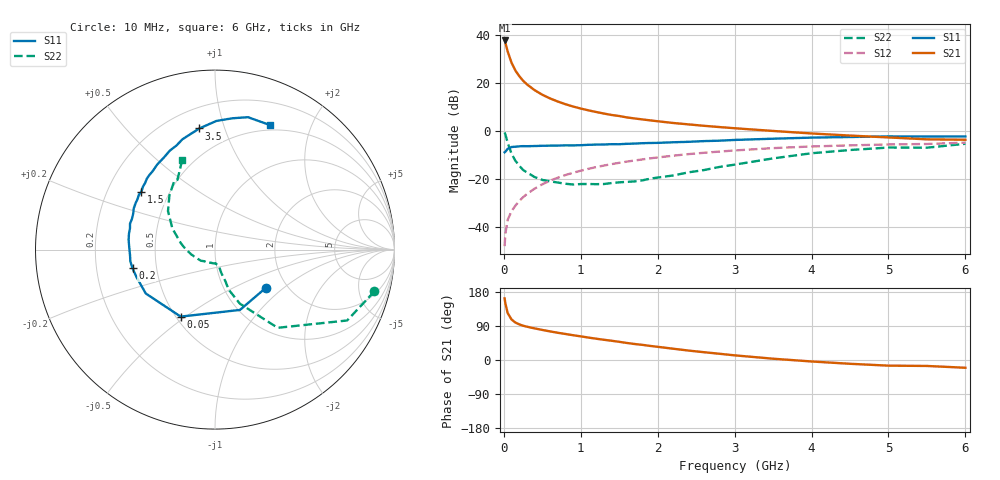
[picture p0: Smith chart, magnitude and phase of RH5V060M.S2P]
! SIEMENS Small Signal Semiconductors
! BFR106
! Si NPN RF Bipolar Junction Transistor in SOT23
! VCE = 5 V  IC = 60 mA
! Common Emitter S-Parameters:  August  1996
# GHz  S  MA  R  50
!  f  S11  S21  S12  S22
! GHz  MAG  ANG  MAG  ANG  MAG  ANG  MAG  ANG
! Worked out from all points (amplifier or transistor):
!   36 points, 10 MHz to 6 GHz, reference 50 ohm
!   highest |S21| = 37.6 dB at 10 MHz (marker M1)
!   |S21| within 3 dB of that: start of sweep to 36.78 MHz
!   unconditionally stable (mu >= 1): 234.5 MHz to 2.299 GHz
!   at 250 MHz: K = 1.01, MAG = 23.6 dB, |S12| = -27.8 dB
!   at 1.4 GHz: K = 1.05, MAG = 8.8 dB, |S12| = -14.0 dB
!   at 6 GHz: K = 0.99, MSG = 0.6 dB, |S12| = -5.0 dB
!   S11 on the Smith chart (normalised r, x): 10 MHz: 1.56, -0.76; 50 MHz: 0.53, -0.48; 200 MHz: 0.36, -0.10; 1.5 GHz: 0.35, +0.31; 3.5 GHz: 0.33, +0.82; 6 GHz: 0.44, +1.44
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0.01  0.3543 -37.0  76.22 162.7  0.0039 83.4  0.9181 -14.7
0.02  0.3638 -67.5  68.27 149.2  0.0072 71.1  0.8356 -28.2
0.05  0.4194 -117.1  44.83 123.8  0.0138 63.0  0.5583 -51.3
0.1  0.4566 -147.6  26.16 106.9  0.0209 62.0  0.3313 -65.3
0.15  0.4632 -160.5  18.01 98.8  0.0273 65.8  0.2363 -71.1
0.2  0.4711 -167.2  13.76 94.1  0.0341 68.4  0.1863 -71.8
0.25  0.4762 -172.2  11.03 90.5  0.0409 70.3  0.1516 -73.6
0.3  0.4744 -176.2  9.257 87.9  0.0478 71.8  0.1347 -74.9
0.4  0.4784 178.1  7.001 83.4  0.0618 72.5  0.1079 -76.0
0.5  0.4842 173.6  5.62 79.3  0.0761 72.6  0.094 -76.9
0.6  0.4874 169.7  4.713 75.5  0.0906 72.0  0.0877 -79.0
0.7  0.4884 165.9  4.065 71.9  0.1043 71.3  0.083 -82.9
0.9  0.4935 159.6  3.192 65.4  0.1326 68.8  0.0754 -88.6
1.1  0.5077 153.1  2.653 59.2  0.1601 66.4  0.0773 -99.2
1.5  0.5217 141.8  2.022 48.0  0.2136 60.8  0.0837 -119.6
1.7  0.5382 136.3  1.798 42.2  0.2388 57.9  0.0874 -131.9
2.2  0.5733 124.1  1.448 29.8  0.3008 50.4  0.1163 -157.7
2.8  0.6184 110.3  1.191 16.5  0.3665 41.2  0.175 175.0
3.5  0.6804 97.4  0.987 3.4  0.4328 30.8  0.2646 153.7
4.5  0.7379 82.5  0.791 -10.0  0.494 16.2  0.3952 130.0
5.5  0.7564 70.3  0.66 -15.7  0.5279 6.6  0.4416 118.3
6  0.7587 66.2  0.647 -20.5  0.5628 -0.6  0.533 110.0
